(* Logix 5000 AddOnInstructionDefinition export Banner_Q90R2KU_PD_v4; software revision 33.00 *)

TYPE Banner_Q90R2KU_PDI0_v4 :   // Process Data for a Q90R2 Analog sensors. Digital Measurement Sensor data set.
STRUCT
   SSC1_State : SINT;   // 0=Inactive, 1=Active
   SSC1_Stability : SINT;   // 0=No target or Marginal, 1=Valid
   AO1_State : SINT;   // 0=Inactive, 1=Active
   AO1_Stability : SINT;   // 0=No target or Marginal, 1=Valid
   SSC1_Distance : DINT;
   SSC1_Beam_Angle : DINT;
   SSC1_Velocity : DINT;
   SSC1_Signal_Strength : INT;
   AO1_Distance : DINT;
   AO1_Beam_Angle : INT;
   AO1_Velocity : DINT;
   AO1_Signal_Strength : INT;
END_STRUCT
END_TYPE

TYPE Banner_Q90R2KU_PDI1_v4 :   // Process Data for a Q90R2 Analog sensors. Distance and Excess Gain data set.
STRUCT
   SSC1_State : SINT;   // 0=Inactive, 1=Active
   SSC1_Stability : SINT;   // 0=No Target or Marginal, 1=Valid
   AO1_State : SINT;   // 0=Inactive, 1=Active
   AO1_Stability : SINT;   // 0=No Target or Marginal, 1=Valid
   SSC1_X : DINT;
   SSC1_Y : DINT;
   SSC1_Velocity : DINT;
   SSC1_Signal_Strength : INT;
   AO1_X : DINT;
   AO1_Y : DINT;
   AO1_Velocity : DINT;
   AO1_Signal_Strength : INT;
END_STRUCT
END_TYPE

TYPE Banner_Q90R2KU_PDI_v4 :   // Process Data for a Q90R2 Analog sensors.
STRUCT
   Set_0 : Banner_Q90R2KU_PDI0_v4;
   Set_1 : Banner_Q90R2KU_PDI1_v4;
   PDI_DT : SINT[16];
END_STRUCT
END_TYPE

ADD_ON_INSTRUCTION Banner_Q90R2KU_PD_v4   (* revision 4.0, vendor Banner Engineering *)
// Take raw process data and convert it to usable values.
VAR_IN_OUT
   PD : Banner_Q90R2KU_PDI_v4; {required}
END_VAR
VAR_INPUT
   Process_Data_Layout : SINT; {required}
   Byte_Swap : BOOL; {required}
END_VAR
VAR
   Temp : SINT[16]; {access None}
END_VAR

ROUTINE Logic   (* ladder *)
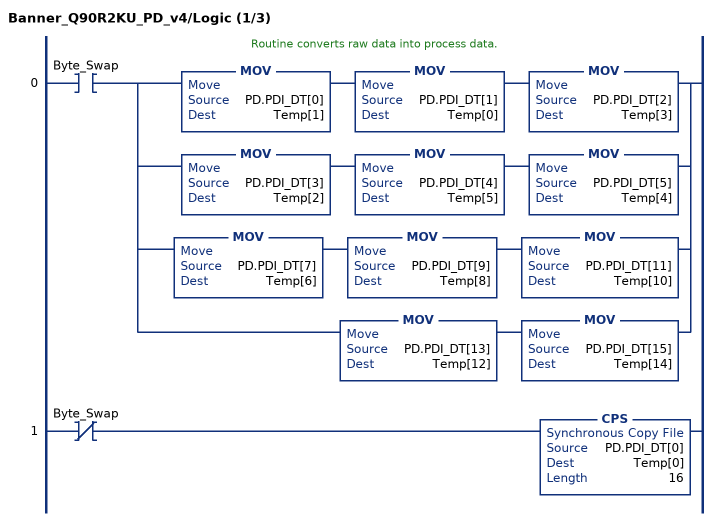
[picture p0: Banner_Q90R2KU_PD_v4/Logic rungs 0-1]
   // Routine converts raw data into process data.
   0: XIC(Byte_Swap)[MOV(PD.PDI_DT[0],Temp[1]) MOV(PD.PDI_DT[1],Temp[0]) MOV(PD.PDI_DT[2],Temp[3]) ,MOV(PD.PDI_DT[3],Temp[2]) MOV(PD.PDI_DT[4],Temp[5]) MOV(PD.PDI_DT[5],Temp[4]) ,MOV(PD.PDI_DT[7],Temp[6]) MOV(PD.PDI_DT[9],Temp[8]) MOV(PD.PDI_DT[11],Temp[10]) ,MOV(PD.PDI_DT[13],Temp[12]) MOV(PD.PDI_DT[15],Temp[14]) ];
   1: XIO(Byte_Swap)CPS(PD.PDI_DT[0],Temp[0],16);
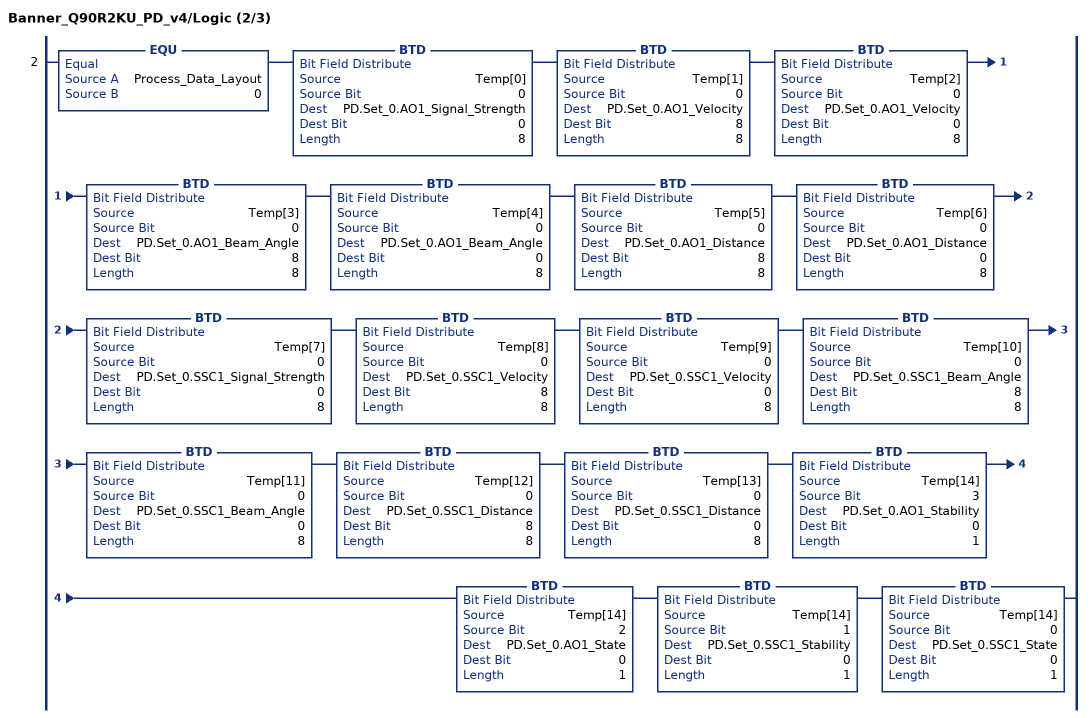
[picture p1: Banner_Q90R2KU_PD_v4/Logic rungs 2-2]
   2: EQU(Process_Data_Layout,0)BTD(Temp[0],0,PD.Set_0.AO1_Signal_Strength,0,8)BTD(Temp[1],0,PD.Set_0.AO1_Velocity,8,8)BTD(Temp[2],0,PD.Set_0.AO1_Velocity,0,8)BTD(Temp[3],0,PD.Set_0.AO1_Beam_Angle,8,8)BTD(Temp[4],0,PD.Set_0.AO1_Beam_Angle,0,8)BTD(Temp[5],0,PD.Set_0.AO1_Distance,8,8)BTD(Temp[6],0,PD.Set_0.AO1_Distance,0,8)BTD(Temp[7],0,PD.Set_0.SSC1_Signal_Strength,0,8)BTD(Temp[8],0,PD.Set_0.SSC1_Velocity,8,8)BTD(Temp[9],0,PD.Set_0.SSC1_Velocity,0,8)BTD(Temp[10],0,PD.Set_0.SSC1_Beam_Angle,8,8)BTD(Temp[11],0,PD.Set_0.SSC1_Beam_Angle,0,8)BTD(Temp[12],0,PD.Set_0.SSC1_Distance,8,8)BTD(Temp[13],0,PD.Set_0.SSC1_Distance,0,8)BTD(Temp[14],3,PD.Set_0.AO1_Stability,0,1)BTD(Temp[14],2,PD.Set_0.AO1_State,0,1)BTD(Temp[14],1,PD.Set_0.SSC1_Stability,0,1)BTD(Temp[14],0,PD.Set_0.SSC1_State,0,1);
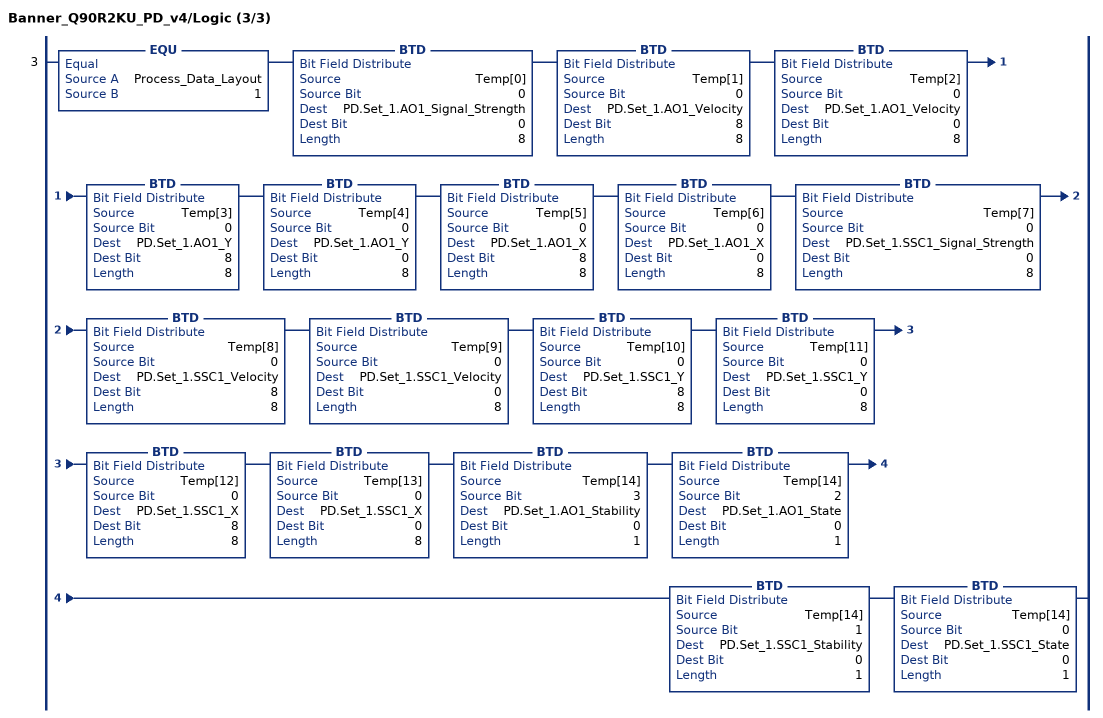
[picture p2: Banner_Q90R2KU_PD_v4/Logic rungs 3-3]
   3: EQU(Process_Data_Layout,1)BTD(Temp[0],0,PD.Set_1.AO1_Signal_Strength,0,8)BTD(Temp[1],0,PD.Set_1.AO1_Velocity,8,8)BTD(Temp[2],0,PD.Set_1.AO1_Velocity,0,8)BTD(Temp[3],0,PD.Set_1.AO1_Y,8,8)BTD(Temp[4],0,PD.Set_1.AO1_Y,0,8)BTD(Temp[5],0,PD.Set_1.AO1_X,8,8)BTD(Temp[6],0,PD.Set_1.AO1_X,0,8)BTD(Temp[7],0,PD.Set_1.SSC1_Signal_Strength,0,8)BTD(Temp[8],0,PD.Set_1.SSC1_Velocity,8,8)BTD(Temp[9],0,PD.Set_1.SSC1_Velocity,0,8)BTD(Temp[10],0,PD.Set_1.SSC1_Y,8,8)BTD(Temp[11],0,PD.Set_1.SSC1_Y,0,8)BTD(Temp[12],0,PD.Set_1.SSC1_X,8,8)BTD(Temp[13],0,PD.Set_1.SSC1_X,0,8)BTD(Temp[14],3,PD.Set_1.AO1_Stability,0,1)BTD(Temp[14],2,PD.Set_1.AO1_State,0,1)BTD(Temp[14],1,PD.Set_1.SSC1_Stability,0,1)BTD(Temp[14],0,PD.Set_1.SSC1_State,0,1);
END_ROUTINE
END_ADD_ON_INSTRUCTION
